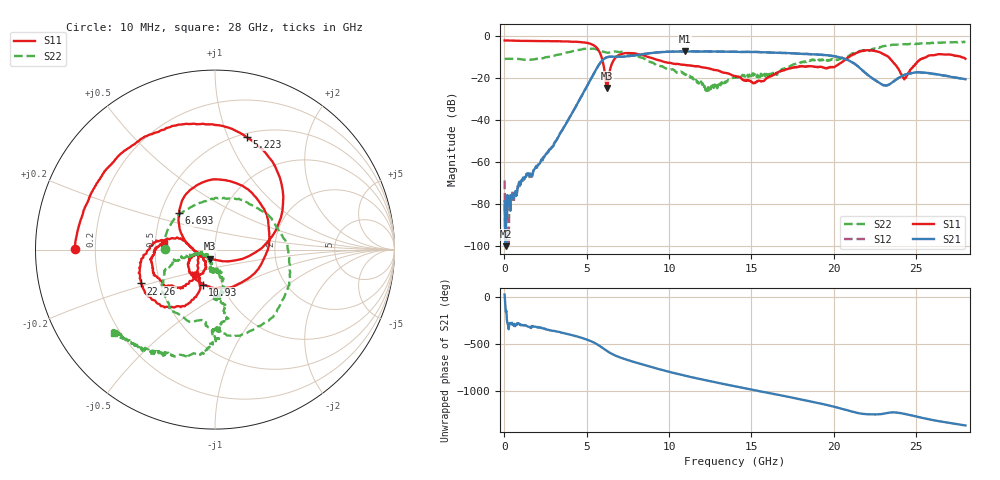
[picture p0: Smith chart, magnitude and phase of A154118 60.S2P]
!  2-Port S-parameters saved by WinCal
! VAR MeasName=S-Parameters (CALIBRATED_DATA) read from VNA (N5230A)
! VAR MeasDate=2015-9-10 14:39:43
! VAR NAME=A154118 60
! VAR FILENAME=A154118 60.S2P
! VAR DATE=2015-9-10 14:39:43
! VAR PHYS_PORTS=1,2
# Hz S DB R 50
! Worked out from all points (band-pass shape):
!   801 points, 10 MHz to 28 GHz, reference 50 ohm
!   highest |S21| = -7.38 dB at 10.96 GHz (marker M1); lowest = -100.2 dB at 79.97 MHz (marker M2)
!   |S21| within 3 dB of the highest: 6.156 GHz to 20.47 GHz (14.31 GHz wide, 107 % of centre)
!   lowest |S11| = -24.8 dB at 6.238 GHz (marker M3), VSWR 1.12, Z = 47.1 - j4.79 ohm
!   |S11| at or under -10 dB: 5.896 GHz to 6.789 GHz (893.4 MHz wide, 14.1 % of centre); 8.73 GHz to 20.93 GHz (12.2 GHz wide, 82.2 % of centre); 23.32 GHz to 25.64 GHz (2.312 GHz wide, 9.45 % of centre)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
!   |S22| runs from -26.2 to -2.8 dB; largest |S21 - S12| = 0.0082
!   S11 on the Smith chart (normalised r, x): 10 MHz: 0.12, +0.00; 5.223 GHz: 0.54, +1.17; 6.693 GHz: 0.62, +0.27; 10.93 GHz: 0.81, -0.33; 22.26 GHz: 0.39, -0.19; 28 GHz: 0.56, +0.05
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1e7  -2.15 179.7  -78.74 29.2  -68.83 156.2  -11.04 179.8
7.9975e7  -2.15 178.7  -100.16 -153.0  -78.38 120.7  -10.88 176.5
2.899e8  -2.19 175.7  -76.44 66.8  -83.88 67.1  -10.86 166.5
2.599075e9  -2.44 144.8  -55.65 15.9  -55.65 16.7  -10.04 61.1
4.698325e9  -3.03 98.3  -28.54 -71.4  -28.54 -71.8  -6.39 -41.8
5.223138e9  -3.73 74.2  -20.90 -103.9  -20.92 -104.4  -6.13 -66.9
5.74795e9  -7.25 30.0  -13.63 -152.5  -13.64 -152.6  -6.97 -90.1
6.237775e9  -24.78 -118.4  -10.12 148.1  -10.11 148.1  -7.98 -98.9
6.692612e9  -10.93 134.7  -9.85 104.2  -9.86 104.0  -7.40 -109.5
7.70725e9  -8.22 74.0  -9.53 41.0  -9.54 40.9  -8.53 -142.4
9.351662e9  -11.50 -22.1  -7.83 -41.8  -7.78 -41.7  -14.18 -167.9
1.09261e10  -13.69 -109.2  -7.41 -111.4  -7.37 -111.9  -17.94 -167.1
1.096109e10  -13.83 -109.9  -7.38 -112.8  -7.33 -113.4  -18.38 -165.5
1.236059e10  -15.33 -151.6  -7.41 -166.9  -7.37 -167.3  -24.43 -145.9
1.4005e10  -19.14 -166.3  -7.57 134.1  -7.57 133.5  -19.83 -104.1
1.585934e10  -20.62 -125.8  -7.81 69.3  -7.74 68.8  -19.38 -94.1
1.869332e10  -14.39 -132.5  -8.74 -29.4  -8.77 -30.0  -11.21 -84.8
2.226205e10  -6.86 -155.4  -19.71 -164.2  -19.79 -165.5  -6.72 -92.1
2.334666e10  -10.25 170.5  -23.19 -146.7  -23.22 -147.2  -4.56 -99.9
2.429132e10  -20.70 -163.5  -18.56 -158.7  -18.61 -159.0  -3.91 -112.2
2.579579e10  -9.36 -143.1  -17.73 143.1  -17.75 142.5  -3.39 -123.7
2.8e10  -10.88 172.4  -20.59 77.9  -20.66 77.3  -2.76 -140.6
